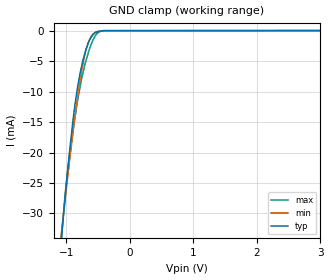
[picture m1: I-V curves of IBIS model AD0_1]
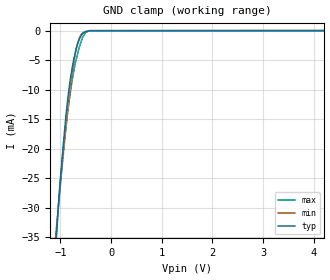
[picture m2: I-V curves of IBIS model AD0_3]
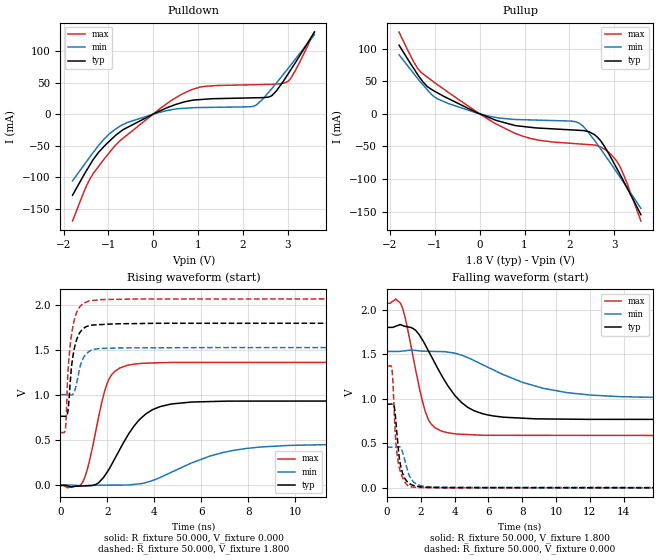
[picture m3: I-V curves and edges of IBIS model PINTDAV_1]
|Texas Instruments Incorporated
|1.2V to 3.6V, 12-Bit, Nanopower, 4-Wire
|TOUCH SCREEN CONTROLLER with I2C Interface
| Marketing part#   Digital Voltage Range   Package-type   #pins
|TSC2014IYZGT   1.2V - 3.6V   3X4 Matrix, 1.5X2.0, WCSP   12-pins
|TSC2014IYZGR   1.2V - 3.6V   3X4 Matrix, 1.5X2.0, WCSP   12-pins
[IBIS Ver]   4.0
[File name]   tsc2014.ibs
[File Rev]   4.0
[Date]   03/17/2010
[Source]   Texas Instruments Incorporated.
   Analog-eLab, HPA
   12500 TI Blvd
   Dallas, TX -75243
   For Support e-mail: elab_ibis@list.ti.com
[Notes]   Revision History:
   1.0: 03/11/2010
   - Initial version of the model
   - Initial Model generated from simulations in TISPICED
   - Model names with a trailing _1 contains the model for
   1.8V (1.53V and 2.07V, +/- 15%). Model names with trailing _3
   contains the model for 3V (2.65V and 3.45V, +/- 15%) operation.
   - Model not matched to measurements
   - Ignore warnings related to min and max values of ccomp,
   The device process of these products is CMOS. The ccomp
   values are based on PVT variations as seen in simulations
   2.0: 08/31/2010
   - C_comp although listed in numerical order of value are
   obtained from varying PVT conditions. For PVT conditions
   for each specific value refer the buffer description under
   respective [Model]. IBIS model user is responsible for using
   appropriate C_comp to simulate for Signal Integrity
   - Change TERM model_name to NC. removed TERM [Model]
   - Corrected marketing package designator from the 16 ball,
   YZH to the 12 ball YZG.
   - Changed pin number B2 from signal_name/model_name A0 to
   AD0.
   3.0: 10/03/2010
   - Modified Vinh for 1.8V (1.14V to 1.26V) models per
   product data sheet.
   - Re-ran and replaced SDA_1 and SDA_3 V-t simulations to correct
   leading edge of the minimum rising waveform and to switch rise
   and fall time data.
   - Re-ran amd replaced PINTDAV_1 and PINTDAV_3 to switch rise and fall
   time data.
   4.0: 03/17/2010
   - Modified SDA_1 and SDA_3 data to reflect buffer more closely.
   - WARNING - Combined Pulldown for Model: SDA_3 Minimum data is
   non-monotonic: error is small and verified with SPICE simulation
   - WARNING - Combined Pulldown for Model: SDA_3 Maximum data is
   non-monotonic: error is small and verified with SPICE simulation
[Disclaimer]
 This product is designed as an aid for customers of Texas Instruments.
 No warranties, either expressed or implied, with respect to this third
 party software (if any) or with respect to its fitness for any
 particular purpose is claimed by Texas Instruments or the author. The
 software (if any) is provided solely on an "as is" basis. The entire
 risk as to its quality and performance is with the customer
[Copyright] (C) Copyright 2010 Texas Instruments Incorporated.
   All rights reserved.
|   TSC2014
[Component]   tsc2014
[Manufacturer] TI
[Package]   | WCSP 3X4
| variable   typ   min   max
R_pkg  0.064167   0.007000   0.197000
L_pkg  1.229917nH  0.360000nH  2.206000nH
C_pkg  1.281750pF  0.537000pF  2.122000pF
[Pin] signal_name  model_name  R_pin  L_pin C_pin
A1   AUX   NC   0.058   1.291nH   1.073pF
A2   VDD   POWER   0.024   0.360nH   1.084pF
A3   XP   NC   0.007   0.367nH   0.537pF
B1   _PINTDAV   PINTDAV   0.125   2.206nH   1.593pF
B2   AD0   AD0   0.055   1.440nH   1.521pF
B3   YP   NC   0.065   1.212nH   0.880pF
C1   SDA   SDA   0.117   1.978nH   1.432pF
C2   _RESET   RESET   0.055   1.424nH   1.525pF
C3   XN   NC   0.032   1.285nH   1.579pF
D1   SCL   SCL   0.197   2.106nH   1.423pF
D2   GND   GND   0.026   0.639nH   2.122pF
D3   YN   NC   0.009   0.451nH   0.612pF
|   Model Selectors
[Model Selector]  AD0
AD0_1   1.8V digital Input
AD0_3   3V digital Input
[Model Selector]  PINTDAV
PINTDAV_1  1.8V digital Output
PINTDAV_3  3V digital Output
[Model Selector]  RESET
RESET_1   1.8V digital Input
RESET_3   3V digital Input
[Model Selector]  SCL
SCL_1   1.8V digital Input
SCL_3   3V digital Input
[Model Selector]  SDA
SDA_1  1.8V digital I/O_open_drain
SDA_3  3V digital I/O_open_drain
| Models and submodels in the file (10): AD0_1 (Input), AD0_3 (Input), PINTDAV_1 (Output), PINTDAV_3 (Output), RESET_1 (Input), RESET_3 (Input), SCL_1 (Input), SCL_3 (Input), SDA_1 (I/O_open_drain), SDA_3 (I/O_open_drain)
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|   1.8V AD0 Model
[Model] AD0_1
Model_type Input
Vinl = 0.54
Vinh = 1.26
|   typ   min   max
|   (nom PVT)   (Fast PVT)   (Slow PVT)
C_comp   3.1255860e-12   2.9996430e-12   3.2993050e-12
|Where nom PVT is NOM Process, 1.8V,27C
|   Fast PVT is Strong Process, 2.07V, -40C
|   Slow PVT is Weak Process, 1.53V, 85C
[Model Spec]
Vinl   0.54   0.459   0.621
Vinh   1.26   1.071   1.449
|VINL  0.3 DVDD, VINH  0.7 DVDD
[Voltage Range]   1.8   1.53   2.07
[Temperature Range]   27   85   -40
[Power Clamp Reference]   1.8   1.53   2.07
[GND Clamp Reference]   0   0   0
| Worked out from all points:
|   GND clamp passes 1 mA (typ) near -0.60 V on its own axis
[GND Clamp]
|   Voltage   I(typ)   I(min)   I(max)
-1.8V     -127mA     -105mA     -167.2mA
-1.074V   -33.84mA   -32.94mA   -34.16mA
-1.064V   -32.73mA   -32.06mA   -32.79mA
-985.9mV  -23.82mA   -24.84mA   -23.68mA
-896.4mV  -14.94mA   -16.98mA   -16.57mA
-816mV    -8.925mA   -10.58mA   -11.15mA
-754.3mV  -5.676mA   -6.39mA    -7.718mA
-686.9mV  -3.019mA   -3.062mA   -4.847mA
-616.8mV  -1.271mA   -1.109mA   -2.51mA
-538mV    -324.3uA   -229.6uA   -784.7uA
-410.9mV  -14.45uA   -11.01uA   -21.16uA
3.6V      0A         0A         0A
[POWER Clamp]
|   SCR cell used for ESD function. Effects occurr above VDD x 2
|   Voltage   I(typ)   I(min)   I(max)
-1.8V     0A         0A         0A
0V        0A         0A         0A
3.6V      0A         0A         0A
|   3.0V AD0 Model
[Model] AD0_3
Model_type Input
Vinl = 0.9
Vinh = 2.1
|   typ   min   max
C_comp   2.7980830e-12   2.6892840e-12   2.9495540e-12
|Where nom PVT is NOM Process, 3V,27C
|   Fast PVT is Strong Process, 3.45V, -40C
|   Slow PVT is Weak Process, 2.65V, 85C
[Model Spec]
Vinl   0.9   0.795   1.035
Vinh   2.1   1.855   2.415
| VINL  0.3 DVDD, VINH  0.7 DVDD
[Voltage Range]   3   2.65   3.45
[Temperature Range]   27   85   -40
[Power Clamp Reference]   3   2.65   3.45
[GND Clamp Reference]   0   0   0
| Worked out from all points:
|   GND clamp passes 1 mA (typ) near -0.60 V on its own axis
[GND Clamp]
|   Voltage   I(typ)   I(min)   I(max)
-3V       -288mA     -228.6mA   -402.1mA
-1.088V   -35.53mA   -34.31mA   -36.22mA
-1.071V   -33.47mA   -32.69mA   -33.78mA
-1.003V   -25.75mA   -26.45mA   -25.41mA
-945.3mV  -19.58mA   -21.22mA   -20.21mA
-879.3mV  -13.49mA   -15.59mA   -15.35mA
-797.3mV  -7.828mA   -9.255mA   -10.04mA
-689.8mV  -3.118mA   -3.175mA   -4.977mA
-623.1mV  -1.37mA    -1.231mA   -2.736mA
-553.3mV  -455.2uA   -323.8uA   -1.027mA
-419.9mV  -16.89uA   -19.58uA   -28.78uA
6V        0A         0A         0A
[POWER Clamp]
|   SCR cell used for ESD function. Effects occurr above VDD x 2
|   Voltage   I(typ)   I(min)   I(max)
-3V       0A         0A         0A
0V        0A         0A         0A
6V        0A         0A         0A
|   1.8V PINTDAV Model
[Model] PINTDAV_1
Model_type Output
Polarity   Non-Inverting
Enable   Active-Low
Vmeas = 0.9
Vref = 0.9
Cref = 15pF
Rref = 50
|   typ   min   max
|   C_comp average
C_comp   8.8520340E-12   8.8153380E-12   9.8123660E-12
|   C_comp high output
|C_comp   1.0339200e-11   1.0133100e-11   1.0637090e-11
|   C_comp low output
|C_comp   7.2914760e-12   7.0669780e-12   9.4916320e-12
|Where nom PVT is NOM Process, 1.8V,27C
|   Fast PVT is Strong Process, 2.07V, -40C
|   Slow PVT is Weak Process, 1.53V, 85C
[Voltage Range]   1.8   1.53   2.07
[Temperature Range]   27   85   -40
[Pullup Reference]   1.8   1.53   2.07
[Pulldown Reference]   0   0   0
[Power Clamp Reference]   1.8   1.53   2.07
[GND Clamp Reference]   0   0   0
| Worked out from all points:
|   slope of the pulldown table from 0 to 0.27 V, typ, clamps not added: 29.9 ohm
|   slope of the pullup table from 0 to 0.27 V, typ, clamps not added: 36.2 ohm
|   falling waveform, R_fixture 50.000, V_fixture 1.800: 20-80 % time 2.03ns typ, 4.19ns min, 996ps max; typ from 1.8 V to 0.768 V
|   rising waveform, R_fixture 50.000, V_fixture 0.000: 20-80 % time 1.36ns typ, 2.65ns min, 702ps max; typ from 0 V to 0.938 V
|   rising waveform, R_fixture 50.000, V_fixture 1.800: 20-80 % time 290ps typ, 326ps min, 273ps max; typ from 0.768 V to 1.8 V
|   falling waveform, R_fixture 50.000, V_fixture 0.000: 20-80 % time 364ps typ, 467ps min, 307ps max; typ from 0.938 V to 0 V
[Pulldown]
|   Voltage   I(typ)   I(min)   I(max)
-1.8V     -128.9mA   -106.1mA   -169.8mA
-1.433V   -83.16mA   -70.05mA   -105.7mA
-1.105V   -52.03mA   -40.43mA   -72.32mA
-715.1mV  -26.97mA   -18.02mA   -40.75mA
138.2mV   4.701mA    2.731mA    7.978mA
629.6mV   18.06mA    8.923mA    31.34mA
1.037V    23.02mA    10.43mA    42.81mA
2.228V    25.83mA    12.25mA    46.66mA
2.64V     29.1mA     40.01mA    47.31mA
2.874V    49.46mA    60.69mA    48.7mA
3.057V    69.24mA    77mA       55.87mA
3.595V    130.3mA    126.3mA    130.4mA
[Pullup]
|   Voltage   I(typ)   I(min)   I(max)
-1.8V     105.5mA    90.84mA    125.7mA
-1.478V   70.19mA    62.45mA    80.53mA
-1.317V   53.9mA     48.61mA    64.26mA
-949.3mV  32.6mA     23.33mA    45.15mA
339.9mV   -9.16mA    -5.178mA   -14.51mA
1.142V    -20.66mA   -9.258mA   -37.86mA
2.148V    -24.94mA   -12.19mA   -45.71mA
2.301V    -25.53mA   -18.7mA    -46.47mA
2.552V    -31.53mA   -39.99mA   -47.71mA
2.829V    -55.32mA   -66.92mA   -56.21mA
3.083V    -87mA      -92.47mA   -75.35mA
3.595V    -154.7mA   -145mA     -164.4mA
[Ramp]
R_load = 50
|   typ   min   max
dV/dt_r   0.562524/1.35293e-009  0.276372/2.63045e-009   0.81965/6.97964e-010
dV/dt_f   0.619399/2.01548e-009  0.313041/4.14874e-009  0.889898/9.92453e-010
[Falling Waveform]
R_fixture = 50.000
V_fixture = 1.800
V_fixture_min = 1.530
V_fixture_max = 2.070
C_fixture = 0.000
|  time   V(typ)   V(min)   V(max)
0s        1.8V       1.53V      2.07V
517.1ps   1.813V     1.53V      2.12V
865ps     1.826V     1.533V     2.045V
1.681ns   1.77V      1.542V     1.339V
2.252ns   1.609V     1.533V     866.5mV
3.181ns   1.279V     1.529V     640.3mV
4.402ns   958.6mV    1.489V     601.2mV
6.286ns   806.8mV    1.324V     589.5mV
10.7ns    770.6mV    1.067V     588.7mV
20ns      767.7mV    1.008V     586.8mV
[Rising Waveform]
R_fixture = 50.000
V_fixture = 0.000
V_fixture_min = 0.000
V_fixture_max = 0.000
C_fixture = 0.000
|  time   V(typ)   V(min)   V(max)
0s        59.19nV    4.695mV    45.54nV
942.3ps   -5.83mV    -4.664mV   34.49mV
1.235ns   -3.289mV   -164.7uV   271.4mV
1.989ns   148.5mV    2.724mV    1.133V
2.297ns   289.2mV    3.252mV    1.262V
2.852ns   549.2mV    4.203mV    1.333V
3.9ns     837.5mV    52.76mV    1.359V
5.593ns   925.2mV    250.3mV    1.365V
8.594ns   935.5mV    427.5mV    1.365V
20ns      937.5mV    456.2mV    1.366V
[Rising Waveform]
R_fixture = 50.000
V_fixture = 1.800
V_fixture_min = 1.530
V_fixture_max = 2.070
C_fixture = 0.000
|  time   V(typ)   V(min)   V(max)
0s        767.7mV    1.008V     586.8mV
216.2ps   766mV      1.006V     637.5mV
246.4ps   767mV      1.006V     760mV
301.6ps   798.3mV    1.005V     1.157V
356.3ps   922.9mV    1.004V     1.392V
464ps     1.299V     1.003V     1.657V
566.7ps   1.488V     1.026V     1.813V
913.5ps   1.728V     1.38V      2.006V
1.235ns   1.773V     1.49V      2.049V
20ns      1.8V       1.53V      2.07V
[Falling Waveform]
R_fixture = 50.000
V_fixture = 0.000
V_fixture_min = 0.000
V_fixture_max = 0.000
C_fixture = 0.000
|  time   V(typ)   V(min)   V(max)
0s        937.5mV    456.2mV    1.366V
304.7ps   940.6mV    456.1mV    1.316V
421.8ps   917.8mV    456.1mV    890.2mV
504.5ps   794.2mV    456.7mV    571.3mV
688.8ps   406.8mV    460.9mV    266.4mV
937.1ps   158mV      392.7mV    110.4mV
1.343ns   46.84mV    128.6mV    15.06mV
1.967ns   12.07mV    25.83mV    3.672mV
3.017ns   2.99mV     8.269mV    1.53mV
20ns      60.09nV    4.695mV    28.46nV
